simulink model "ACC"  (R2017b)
settings: Solver=FixedStepDiscrete  StartTime=0.0  StopTime=10.0  FixedStep=0.01  RelTol=1e-3  EnableMultiTasking=on
undefined symbols (not defined in the file): ACC_CONST0_NUMB, ACC_CONST1000_NUMB, ACC_CONST100_NUMB, ACC_CONST121_NUMB, ACC_CONST1_NUMB, ACC_CONST2047_NUMB, ACC_CONST60000_NUMB, ACC_CONST60_NUMB, ACC_CONSTF1_NUMB, ACC_RUNTIME_MS, ASWTYPE_FALSE, ASWTYPE_TRUE, CcACC_ACChrgDispSOCPrmt_pct, CcACC_ACChrgMismatch_ms, CcACC_ACChrgPACKVolLim_V, CcACC_ACChrgPACKVolLimTi_ms, CcACC_ACChrgPrmtObcFltLvl_numb, CcACC_ACChrgPrmtVcuFltLvl_numb, CcACC_ACChrgStepCurr_A, CcACC_ACChrgTempPrmtDelayTime_ms, CcACC_ACCrntUnctrolTi_ms, CcACC_ACFullChrgHysVolt_mV, CcACC_ACFullStepChrgTi1_ms, CcACC_ACFullStepChrgTi2_ms, CcACC_ACMaxChrgCurr_A, CcACC_ACStepChrgWaitTime_ms, CcACC_ACStop2DefaultTi_ms, CcACC_ACStop2DefaultTiDelay_ms, CcACC_BatFullResetTime_ms, CcACC_ChrgCrnt0HysVolt_mV, CcACC_ChrgEndDeviationVol1_mV, CcACC_ChrgEndDeviationVol2_mV, CcACC_ChrgEndDeviationVol3_mV, CcACC_ChrgMaxPackVoltLimt_V, CcACC_ChrgPwr1_W, CcACC_ChrgPwr2_W, CcACC_ChrgPwr3_W, CcACC_ChrgSt2StepChrgDeviVol_mV, CcACC_ChrgSt2StepChrgTime_ms, CcACC_ChrgStCutoffTime_ms, CcACC_ChrgStFullChrgCrnt_A, CcACC_CPDutyLowThrhd_pct, CcACC_CrntFilterTi1_cnt, CcACC_CrntFilterTi2_cnt, CcACC_CrntFilterTi2_ms, CcACC_CurrObcPreHeatLowThrhd_A, CcACC_DiffACChrgCrnt_A, CcACC_DiffACChrgCrntTi_ms, CcACC_DispSOCCalStart_pct, CcACC_DispSOCDiff_pct, CcACC_ElecLckRemTimeHold_ms, CcACC_HeatChrgCrnt0Time_ms, CcACC_HeatChrgCrnt1Time_ms, CcACC_Initial500Ti_ms, CcACC_Initial700Ti_ms, CcACC_MaxACChrgCellTemp_C, CcACC_MaxPackVoltLimt_V, CcACC_MinACChrgCellTemp_C, CcACC_MinACChrgCrntRqst_A, CcACC_OBCChrgPwr_W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
libraries: AIWAYS_Powertrain_BMS_lib x94, simulink x2
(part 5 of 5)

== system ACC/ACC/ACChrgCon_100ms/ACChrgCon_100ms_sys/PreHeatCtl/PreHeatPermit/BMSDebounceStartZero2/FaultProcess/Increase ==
  FaultStep : Inport
  Counter : Inport  Port=2
  Add : Sum  AccumDataTypeStr=uint16  OutDataTypeStr=uint16
  Saturation : Saturate  UpperLimit=60000  LowerLimit=0
  FaultCnt : Outport
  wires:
  Saturation/1 -> FaultCnt/1
  Add/1 -> Saturation/1
  Counter/1 -> Add/2
  FaultStep/1 -> Add/1

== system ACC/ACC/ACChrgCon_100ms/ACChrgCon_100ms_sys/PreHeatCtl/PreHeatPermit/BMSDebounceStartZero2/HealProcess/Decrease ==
  HealStep : Inport
  Counter : Inport  Port=2
  Constant : Constant  Value=0  OutDataTypeStr=Inherit: Inherit via back propagation
  Nomal : Subsystem
  Relational Operator : RelationalOperator  OutDataTypeStr=boolean
  Switch : Switch  Criteria=u2 ~= 0
  HealCnt : Outport
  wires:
  Constant/1 -> Switch/3
  Relational Operator/1 -> Switch/2
  Nomal/1(HealCnt) -> Switch/1
  Switch/1 -> HealCnt/1
  Counter/1 -> Relational Operator/1, Nomal/2(Counter)
  HealStep/1 -> Relational Operator/2, Nomal/1(HealStep)

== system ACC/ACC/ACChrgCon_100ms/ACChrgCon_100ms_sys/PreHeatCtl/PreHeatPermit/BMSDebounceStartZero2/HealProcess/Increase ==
  HealStep : Inport
  Counter : Inport  Port=2
  Add : Sum  AccumDataTypeStr=uint16  OutDataTypeStr=uint16
  Saturation : Saturate  UpperLimit=60000  LowerLimit=0
  HealCnt : Outport
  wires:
  HealStep/1 -> Add/1
  Counter/1 -> Add/2
  Add/1 -> Saturation/1
  Saturation/1 -> HealCnt/1

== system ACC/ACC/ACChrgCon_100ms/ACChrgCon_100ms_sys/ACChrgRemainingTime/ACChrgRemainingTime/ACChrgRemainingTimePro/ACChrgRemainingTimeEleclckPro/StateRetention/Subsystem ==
  clear : Inport
  set : Inport  Port=2
  Logical Operator1 : Logic  AllPortsSameDT=off  OutDataTypeStr=boolean
  Logical Operator2 : Logic  Operator=OR  AllPortsSameDT=off  OutDataTypeStr=boolean
  Logical2 : Logic  Operator=NOT  OutDataTypeStr=boolean
  Unit Delay1 : UnitDelay  SampleTime=-1  StateName=StateName
  Q : Outport
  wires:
  set/1 -> Logical Operator2/2
  Logical Operator1/1 -> Q/1, Unit Delay1/1
  Logical Operator2/1 -> Logical Operator1/1
  clear/1 -> Logical2/1
  Unit Delay1/1 -> Logical Operator2/1
  Logical2/1 -> Logical Operator1/2

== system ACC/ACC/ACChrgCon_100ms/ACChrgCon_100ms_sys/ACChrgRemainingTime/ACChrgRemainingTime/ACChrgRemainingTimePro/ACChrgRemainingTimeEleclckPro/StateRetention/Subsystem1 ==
  En : Inport
  Ts : Inport  Port=2
  Rst : Inport  Port=3
  Vst : Inport  Port=4
  Constant2 : Constant  Value=ACC_CONST0_NUMB
  Data Type Conversion1 : DataTypeConversion
  Sum2 : Sum  OutDataTypeStr=Inherit: Inherit via back propagation  RndMeth=Zero
  Switch1 : Switch  Criteria=u2 ~= 0
  Switch2 : Switch  Criteria=u2 ~= 0
  Unit Delay1 : UnitDelay  SampleTime=-1  StateName=StateName
  Timer : Outport
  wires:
  Vst/1 -> Switch1/1
  Rst/1 -> Switch1/2
  Ts/1 -> Switch2/1
  En/1 -> Switch2/2
  Switch2/1 -> Sum2/1
  Unit Delay1/1 -> Sum2/2
  Sum2/1 -> Switch1/3
  Switch1/1 -> Unit Delay1/1, Timer/1
  Constant2/1 -> Data Type Conversion1/1
  Data Type Conversion1/1 -> Switch2/3

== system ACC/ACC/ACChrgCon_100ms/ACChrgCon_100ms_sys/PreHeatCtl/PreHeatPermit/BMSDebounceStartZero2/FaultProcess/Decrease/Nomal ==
  FaultStep : Inport
  Counter : Inport  Port=2
  Add : Sum  Inputs=+-  AccumDataTypeStr=uint16  OutDataTypeStr=uint16
  FaultCnt : Outport
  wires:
  Add/1 -> FaultCnt/1
  FaultStep/1 -> Add/2
  Counter/1 -> Add/1

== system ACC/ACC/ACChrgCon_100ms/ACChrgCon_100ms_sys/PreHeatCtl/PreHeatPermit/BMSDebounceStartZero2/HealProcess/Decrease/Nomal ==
  HealStep : Inport
  Counter : Inport  Port=2
  Add : Sum  Inputs=+-  AccumDataTypeStr=uint16  OutDataTypeStr=uint16
  HealCnt : Outport
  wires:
  Counter/1 -> Add/1
  HealStep/1 -> Add/2
  Add/1 -> HealCnt/1

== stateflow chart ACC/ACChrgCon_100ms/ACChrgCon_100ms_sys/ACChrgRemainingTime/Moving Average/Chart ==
  (default) -> (junction 16)
  (junction 16) -> (junction 17) : [R]
  (junction 16) -> (junction 18)
  (junction 17) -> (junction 22) : {count = 0;...  sum = 0;...  buffer = 0;...  average = 0;...  index = 0;}
  (junction 18) -> (junction 19) : [count >= BufferSize]
  (junction 18) -> (junction 21) : {count = count +1;}
  (junction 19) -> (junction 20) : {sum = sum - buffer[index];}
  (junction 20) -> (junction 21)
  (junction 21) -> (junction 25) : {sum = sum + u;... buffer[index] =u;... average = sum/count;}
  (junction 25) -> (junction 24) : [index >= BufferSize-1]
  (junction 25) -> (junction 26) : {index = index+1;}
  (junction 24) -> (junction 27) : {index = 0;}
  (junction 27) -> (junction 26)
  (junction 22) -> (junction 27)
  (junction 26) -> (junction 23) : {Y=average;}
  data: count local uint16 [0..500]; buffer local single; u input single; index local uint16 [0..499]; R input boolean; sum local single; BufferSize parameter uint16 [1..500]; Y output single; average local single

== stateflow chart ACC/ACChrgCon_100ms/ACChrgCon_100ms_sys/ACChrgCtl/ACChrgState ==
  state ACC_ACDefault
    en:
    GeACC_ACChrgState_enum = Enum_ACCACChrgState.Enum_ACCACChrgState_Default;
    LbACC_ObcChrgCmd_flg = ASWTYPE_FALSE;
    GcACC_ACChrgVoltRqst_V = ACC_CONST0_NUMB;
    LcACC_ACChrgCurrRqst_A = ACC_CONST0_NUMB;
    GbACC_ACChrgFinish_flg = ASWTYPE_FALSE;
    GbACC_ACChrgRqst_flg = LbACC_ACChrgPrmt_flg;
    du:
    GbACC_ACChrgCtrCmd_flg =  LbACC_ACChrgPrmt_flg;
    GbACC_ACChrgRqst_flg = LbACC_ACChrgPrmt_flg;
  state ACC_ACChrg
    en:
    GeACC_ACChrgState_enum = Enum_ACCACChrgState.Enum_ACCACChrgState_Chrg;
    GcACC_ACChrgVoltRqst_V = CcACC_ChrgMaxPackVoltLimt_V;
    LcACC_ACChrgCurrRqst_A = GcSOP_MaxChrgCurr_A;
    du:
    LcACC_ACChrgCurrRqst_A = GcSOP_MaxChrgCurr_A;
    LbACC_ObcChrgCmd_flg = ASWTYPE_TRUE;
    ex:
    GbACC_ACChrgFinish_flg = LbACC_FinishInChrgSt_flg;
  state ACC_ACStop
    en:
    GeACC_ACChrgState_enum = Enum_ACCACChrgState.Enum_ACCACChrgState_Stop;
    LbACC_ObcChrgCmd_flg = ASWTYPE_FALSE;
    GcACC_ACChrgVoltRqst_V = ACC_CONST0_NUMB;
    LcACC_ACChrgCurrRqst_A = ACC_CONST0_NUMB;
    GbACC_ACChrgCtrCmd_flg = ASWTYPE_FALSE;
    GbACC_ACChrgRqst_flg = ASWTYPE_FALSE;
  state ACC_ACStepChrg
    en:
    GeACC_ACChrgState_enum = Enum_ACCACChrgState.Enum_ACCACChrgState_StepChrg;
    GcACC_ACChrgVoltRqst_V = CcACC_ChrgMaxPackVoltLimt_V;
    LbACC_ObcChrgCmd_flg = ASWTYPE_TRUE;
    du:
    LcACC_ACChrgCurrRqst_A = GcSOP_MaxChrgCurr_A;
    LbACC_ObcChrgCmd_flg = ASWTYPE_TRUE;
    ex:
    GbACC_ACChrgFinish_flg = LbACC_FinishInStepChrg_flg;
  (default) -> ACC_ACDefault
  ACC_ACStop -> ACC_ACDefault : [ASWTYPE_TRUE == LbACC_Stop2Default_flg]
  ACC_ACDefault -> ACC_ACChrg : [ASWTYPE_TRUE == LbACC_ChrgStateDef2Chrg_flg]
  ACC_ACChrg -> ACC_ACStop : [ASWTYPE_TRUE == LbACC_ChrgSt2Stop_flg]
  ACC_ACChrg -> ACC_ACStepChrg : [ASWTYPE_TRUE == LbACC_ChrgSt2StepChrg_flg]
  ACC_ACStepChrg -> ACC_ACStop : [ASWTYPE_TRUE== LbACC_StepChrg2Stop_flg]
  data: GeACC_ACChrgState_enum output; LcACC_ACChrgCurrRqst_A output; GcACC_ACChrgVoltRqst_V output; LbACC_ChrgStateDef2Chrg_flg input; CcACC_ChrgMaxPackVoltLimt_V parameter; ACC_CONST0_NUMB parameter; LbACC_ChrgSt2StepChrg_flg input; LbACC_ChrgSt2Stop_flg input; LbACC_FinishInChrgSt_flg input; LcACC_StepChrgCrntReq_A input; LbACC_StepChrg2Stop_flg input; LbACC_FinishInStepChrg_flg input; ASWTYPE_TRUE parameter; GbACC_ACChrgPrmt_flg input; GcSOP_MaxChrgCurr_A input; GbACC_ACChrgCtrCmd_flg output; GbACC_ACChrgFinish_flg output; ASWTYPE_FALSE parameter; GbACC_ACChrgRqst_flg output; LbACC_ObcChrgCmd_flg output; LbACC_ACChrgPrmt_flg input; LbACC_Stop2Default_flg input

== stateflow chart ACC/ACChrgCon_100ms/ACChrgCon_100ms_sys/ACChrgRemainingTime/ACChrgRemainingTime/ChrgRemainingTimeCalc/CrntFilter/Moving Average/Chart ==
  (default) -> (junction 16)
  (junction 16) -> (junction 17) : [R]
  (junction 16) -> (junction 18)
  (junction 17) -> (junction 22) : {count = 0;...  sum = 0;...  buffer = 0;...  average = 0;...  index = 0;}
  (junction 18) -> (junction 19) : [count >= BufferSize]
  (junction 18) -> (junction 21) : {count = count +1;}
  (junction 19) -> (junction 20) : {sum = sum - buffer[index];}
  (junction 20) -> (junction 21)
  (junction 21) -> (junction 25) : {sum = sum + u;... buffer[index] =u;... average = sum/count;}
  (junction 25) -> (junction 24) : [index >= BufferSize-1]
  (junction 25) -> (junction 26) : {index = index+1;}
  (junction 24) -> (junction 27) : {index = 0;}
  (junction 27) -> (junction 26)
  (junction 22) -> (junction 27)
  (junction 26) -> (junction 23) : {Y=average;}
  data: count local uint16 [0..500]; buffer local single; u input single; index local uint16 [0..499]; R input boolean; sum local single; BufferSize parameter uint16 [1..500]; Y output single; average local single
